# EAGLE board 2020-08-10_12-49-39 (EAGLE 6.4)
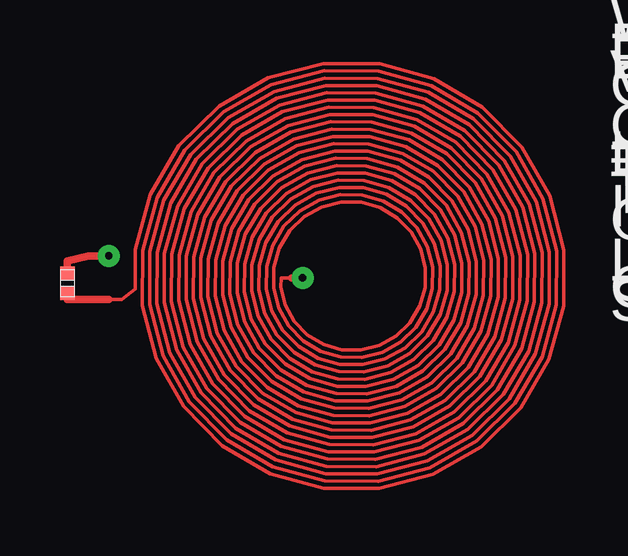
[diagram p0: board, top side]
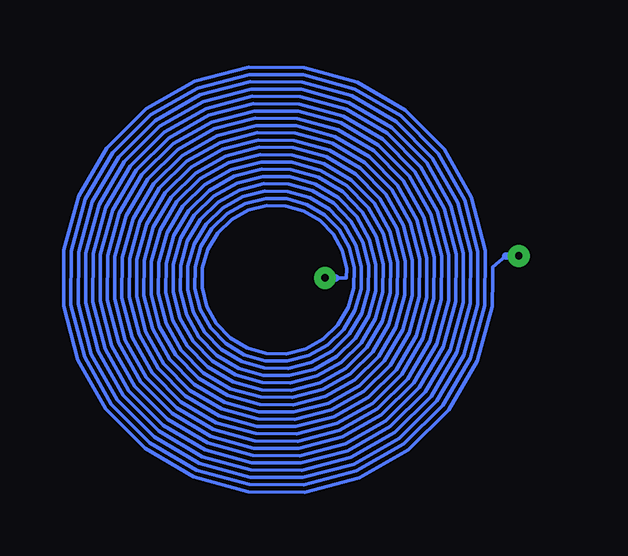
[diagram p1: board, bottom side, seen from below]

No outline drawn. Coordinates in mm, seen from the top.
Copper layers ((1*2)+(15*16)): TOP / INTERNAL1 / layer 15 / BOTTOM

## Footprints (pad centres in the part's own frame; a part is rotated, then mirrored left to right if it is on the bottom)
0402 = smd 0.559 x 0.61: 1 -0.419,0; 2 0.419,0

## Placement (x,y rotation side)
CSensor  [0402]  2.03,12.09 90 top

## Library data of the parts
CSensor = ultra-librarian

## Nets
3: CSensor.1 CSensor.2

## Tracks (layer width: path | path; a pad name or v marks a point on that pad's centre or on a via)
3  (via drill 0.3 pad 0.91)
  TOP 0.152: 11.39,12.32 10.94,12.32 10.93,11.93 11.12,11.18 11.49,10.5 12.04,9.94 12.71,9.53 13.47,9.32 14.26,9.3 15.03,9.5 15.73,9.88 16.31,10.44 16.72,11.13 16.94,11.91 16.95,12.72 16.75,13.51 16.36,14.23 15.79,14.82 15.08,15.24 14.28,15.47 13.45,15.48 12.64,15.28 11.91,14.87 11.3,14.28 10.87,13.56 10.64,12.74 10.62,11.89 10.83,11.06 11.25,10.31 11.85,9.69 12.6,9.25 13.43,9.01 14.3,9 15.15,9.21 15.92,9.64 16.55,10.26 17,11.02 17.25,11.87 17.26,12.76 17.04,13.63 16.6,14.41 15.97,15.06 15.19,15.52 14.32,15.77 13.41,15.78 12.52,15.56 11.72,15.11 11.06,14.47 10.59,13.67 10.33,12.78 10.32,11.85 10.55,10.94 11.01,10.12 11.67,9.45 12.48,8.97 13.39,8.71 14.34,8.7 15.27,8.93 16.1,9.4 16.79,10.07 17.29,10.9 17.55,11.83 17.56,12.8 17.32,13.75 16.84,14.6 16.16,15.3 15.31,15.81 14.36,16.07 13.37,16.09 12.4,15.84 11.53,15.35 10.82,14.65 10.3,13.79 10.03,12.82 10.02,11.81 10.27,10.83 10.77,9.94 11.48,9.21 12.36,8.68 13.35,8.4 14.38,8.39 15.38,8.65 16.29,9.16 17.04,9.88 17.57,10.78 17.85,11.79 17.86,12.84 17.6,13.86 17.09,14.79 16.34,15.55 15.43,16.09 14.4,16.38 13.33,16.39 12.29,16.12 11.35,15.6 10.57,14.84 10.02,13.91 9.73,12.86 9.71,11.77 9.98,10.71 10.52,9.75 11.29,8.96 12.24,8.4 13.31,8.1 14.42,8.09 15.5,8.36 16.48,8.91 17.28,9.7 17.85,10.66 18.16,11.75 18.17,12.88 17.89,13.98 17.33,14.97 16.53,15.79 15.55,16.37 14.44,16.68 13.29,16.7 12.17,16.41 11.16,15.84 10.33,15.03 9.74,14.03 9.42,12.9 9.41,11.73 9.7,10.59 10.28,9.56 11.11,8.72 12.13,8.12 13.27,7.8 14.46,7.78 15.62,8.08 16.66,8.67 17.52,9.51 18.14,10.55 18.46,11.71 18.47,12.92 18.17,14.1 17.57,15.16 16.72,16.03 15.66,16.66 14.48,16.99 13.25,17 12.05,16.69 10.97,16.08 10.09,15.21 9.45,14.14 9.12,12.94 9.11,11.69 9.42,10.47 10.04,9.38 10.92,8.48 12.01,7.83 13.23,7.49 14.5,7.48 15.74,7.8 16.85,8.43 17.77,9.32 18.42,10.43 18.76,11.67 18.78,12.96 18.45,14.22 17.82,15.35 16.9,16.28 15.78,16.94 14.52,17.29 13.21,17.3 11.94,16.97 10.79,16.33 9.84,15.4 9.17,14.26 8.81,12.98 8.8,11.65 9.14,10.36 9.79,9.19 10.73,8.23 11.89,7.55 13.19,7.19 14.54,7.18 15.85,7.51 17.04,8.18 18.01,9.14 18.7,10.31 19.07,11.63 19.08,13 18.74,14.33 18.06,15.53 17.09,16.52 15.9,17.22 14.56,17.59 13.17,17.61 11.82,17.26 10.6,16.57 9.6,15.59 8.89,14.38 8.51,13.02 8.5,11.61 8.85,10.24 9.55,9.01 10.55,7.99 11.77,7.27 13.15,6.89 14.58,6.87 15.97,7.23 17.22,7.94 18.25,8.95 18.98,10.2 19.37,11.59 19.38,13.04 19.02,14.45 18.3,15.72 17.28,16.76 16.02,17.5 14.6,17.9 13.13,17.91 11.7,17.54 10.41,16.81 9.36,15.77 8.61,14.49 8.21,13.06 8.2,11.57 8.57,10.12 9.31,8.82 10.36,7.75 11.66,6.98 13.11,6.58 14.62,6.57 16.09,6.95 17.41,7.7 18.49,8.76 19.27,10.08 19.68,11.55 19.69,13.08 19.3,14.57 18.54,15.91 17.46,17 16.13,17.79 14.64,18.2 13.09,18.21 11.58,17.82 10.23,17.06 9.12,15.96 8.32,14.61 7.9,13.1 7.89,11.53 8.29,10.01 9.06,8.63 10.17,7.5 11.54,6.7 13.07,6.28 14.66,6.27 16.2,6.67 17.6,7.45 18.74,8.58 19.55,9.96 19.98,11.51 19.99,13.12 19.59,14.69 18.79,16.09 17.65,17.25 16.25,18.07 14.68,18.5 13.05,18.52 11.47,18.11 10.04,17.3 8.87,16.15 8.04,14.73 7.6,13.14 7.59,11.49 8,9.89 8.82,8.45 9.99,7.26 11.42,6.42 13.03,5.97 14.7,5.96 16.32,6.38 17.78,7.21 18.98,8.39 19.83,9.84 20.28,11.47 20.3,13.16 19.87,14.8 19.03,16.28 17.84,17.49 16.37,18.36 14.72,18.81 13.01,18.82 11.35,18.39 9.86,17.54 8.63,16.33 7.76,14.85 7.3,13.18 7.28,11.45 7.72,9.77 8.58,8.26 9.8,7.02 11.3,6.13 12.99,5.67 14.74,5.66 16.44,6.1 17.97,6.97 19.22,8.2 20.12,9.73 20.59,11.43 20.6,13.2 20.15,14.92 19.27,16.47 18.02,17.73 16.48,18.64 14.76,19.11 12.97,19.12 11.23,18.67 9.67,17.79 8.39,16.52 7.47,14.96 6.99,13.22 6.98,11.41 7.44,9.65 8.34,8.07 9.61,6.78 11.19,5.85 12.95,5.37 14.78,5.35 16.56,5.82 18.16,6.72 19.47,8.02 20.4,9.61 20.89,11.39 20.9,13.24 20.43,15.04 19.52,16.65 18.21,17.98 16.6,18.92 14.8,19.42 12.93,19.43 11.12,18.96 9.48,18.03 8.14,16.71 7.19,15.08 6.69,13.26 6.68,11.37 7.15,9.54 8.09,7.89 9.43,6.53 11.07,5.57 12.91,5.06 14.82,5.05 16.67,5.53 18.34,6.48 19.71,7.83 20.68,9.49 21.19,11.35 21.21,13.28 20.72,15.15 19.76,16.84 18.4,18.22 16.72,19.2 14.84,19.72 12.89,19.73 11,19.24 9.29,18.27 7.9,16.89 6.91,15.2 6.38,13.3 6.37,11.33 6.87,9.42 7.85,7.7 9.24,6.29 10.95,5.29 12.87,4.76 14.86,4.75 16.79,5.25 18.53,6.24 19.95,7.64 20.97,9.37 21.5,11.31 21.51,13.32 21,15.27 20,17.02 18.58,18.46 16.84,19.49 14.88,20.02 12.85,20.04 10.88,19.52 9.11,18.51 7.66,17.08 6.62,15.31 6.08,13.34 6.07,11.29 6.59,9.3 7.61,7.51 9.05,6.05 10.84,5 12.83,4.46 14.9,4.44 16.91,4.97 18.71,6 20.2,7.46 21.25,9.26 21.8,11.27 21.81,13.36 21.28,15.39 20.25,17.21 18.77,18.71 16.95,19.77 14.92,20.33 12.81,20.34 10.76,19.8 8.92,18.76 7.41,17.27 6.34,15.43 5.78,13.38 5.76,11.25 6.3,9.18 7.36,7.33 8.87,5.8 10.72,4.72 12.79,4.15 14.94,4.14 17.03,4.68 18.9,5.75 20.44,7.27 21.53,9.14 22.11,11.23 22.12,13.4 21.57,15.51 20.49,17.4 18.96,18.95 17.07,20.05 14.96,20.63 12.77,20.64 10.65,20.09 8.74,19 7.17,17.45 6.06,15.55 5.47,13.42 5.46,11.21 6.02,9.07 7.12,7.14 8.68,5.56 10.6,4.44 12.75,3.85 14.98,3.83 17.14,4.4 19.09,5.51 20.68,7.08 21.82,9.02 22.41,11.19 22.42,13.44 21.85,15.62 20.73,17.59 19.14,19.19 17.19,20.34 15,20.93 12.73,20.95 10.53,20.37 8.55,19.24 6.93,17.64 5.77,15.67 5.17,13.46 5.16,11.17 5.74,8.95 6.88,6.95 8.49,5.32 10.48,4.15 12.71,3.54 15.02,3.53 17.26,4.12 19.27,5.27 20.93,6.9 22.1,8.9 22.71,11.15 22.73,13.48 22.13,15.74 20.98,17.77 19.33,19.44 17.3,20.62 15.04,21.24 12.69,21.25 10.41,20.65 8.36,19.49 6.68,17.83 5.49,15.78 4.87,13.5 4.85,12.32 4.85,11.86 4.31,11.4 3.76,11.4
  TOP 0.304: 11.39,12.32 v11.84,12.32 | v3.76,13.23 2.9,13.23 2.03,13.01 2.03,12.8 | 3.76,11.4 2.9,11.4 2.03,11.4
  BOTTOM 0.152: 11.39,12.32 10.94,12.32 10.93,12.7 11.12,13.45 11.49,14.13 12.04,14.7 12.71,15.1 13.47,15.31 14.26,15.33 15.03,15.13 15.73,14.75 16.31,14.19 16.72,13.5 16.94,12.72 16.95,11.91 16.75,11.12 16.36,10.4 15.79,9.81 15.08,9.39 14.28,9.16 13.45,9.15 12.64,9.36 11.91,9.76 11.3,10.35 10.87,11.07 10.64,11.89 10.62,12.74 10.83,13.57 11.25,14.32 11.85,14.94 12.6,15.38 13.43,15.62 14.3,15.63 15.15,15.42 15.92,14.99 16.55,14.38 17,13.62 17.25,12.76 17.26,11.87 17.04,11 16.6,10.22 15.97,9.57 15.19,9.11 14.32,8.86 13.41,8.85 12.52,9.07 11.72,9.52 11.06,10.16 10.59,10.96 10.33,11.85 10.32,12.78 10.55,13.69 11.01,14.51 11.67,15.18 12.48,15.66 13.39,15.92 14.34,15.94 15.27,15.7 16.1,15.23 16.79,14.56 17.29,13.73 17.55,12.8 17.56,11.83 17.32,10.88 16.84,10.03 16.16,9.33 15.31,8.82 14.36,8.56 13.37,8.54 12.4,8.79 11.53,9.28 10.82,9.98 10.3,10.84 10.03,11.81 10.02,12.82 10.27,13.81 10.77,14.69 11.48,15.43 12.36,15.95 13.35,16.23 14.38,16.24 15.38,15.98 16.29,15.48 17.04,14.75 17.57,13.85 17.85,12.84 17.86,11.79 17.6,10.77 17.09,9.84 16.34,9.09 15.43,8.54 14.4,8.25 13.33,8.24 12.29,8.51 11.35,9.03 10.57,9.79 10.02,10.72 9.73,11.77 9.71,12.86 9.98,13.92 10.52,14.88 11.29,15.67 12.24,16.23 13.31,16.53 14.42,16.54 15.5,16.27 16.48,15.72 17.28,14.94 17.85,13.97 18.16,12.88 18.17,11.75 17.89,10.65 17.33,9.66 16.53,8.84 15.55,8.26 14.44,7.95 13.29,7.94 12.17,8.22 11.16,8.79 10.33,9.6 9.74,10.61 9.42,11.73 9.41,12.9 9.7,14.04 10.28,15.07 11.11,15.91 12.13,16.51 13.27,16.83 14.46,16.85 15.62,16.55 16.66,15.96 17.52,15.12 18.14,14.08 18.46,12.92 18.47,11.71 18.17,10.53 17.57,9.47 16.72,8.6 15.66,7.97 14.48,7.64 13.25,7.63 12.05,7.94 10.97,8.55 10.09,9.42 9.45,10.49 9.12,11.69 9.11,12.94 9.42,14.16 10.04,15.25 10.92,16.15 12.01,16.8 13.23,17.14 14.5,17.15 15.74,16.83 16.85,16.2 17.77,15.31 18.42,14.2 18.76,12.96 18.78,11.67 18.45,10.41 17.82,9.29 16.9,8.36 15.78,7.69 14.52,7.34 13.21,7.33 11.94,7.66 10.79,8.3 9.84,9.23 9.17,10.37 8.81,11.65 8.8,12.98 9.14,14.28 9.79,15.44 10.73,16.4 11.89,17.08 13.19,17.44 14.54,17.45 15.85,17.12 17.04,16.45 18.01,15.49 18.7,14.32 19.07,13 19.08,11.63 18.74,10.3 18.06,9.1 17.09,8.11 15.9,7.41 14.56,7.04 13.17,7.03 11.82,7.37 10.6,8.06 9.6,9.04 8.89,10.25 8.51,11.61 8.5,13.02 8.85,14.39 9.55,15.63 10.55,16.64 11.77,17.36 13.15,17.75 14.58,17.76 15.97,17.4 17.22,16.69 18.25,15.68 18.98,14.44 19.37,13.04 19.38,11.59 19.02,10.18 18.3,8.91 17.28,7.87 16.02,7.13 14.6,6.73 13.13,6.72 11.7,7.09 10.41,7.82 9.36,8.86 8.61,10.14 8.21,11.57 8.2,13.06 8.57,14.51 9.31,15.81 10.36,16.88 11.66,17.65 13.11,18.05 14.62,18.06 16.09,17.68 17.41,16.93 18.49,15.87 19.27,14.55 19.68,13.08 19.69,11.55 19.3,10.06 18.54,8.72 17.46,7.63 16.13,6.84 14.64,6.43 13.09,6.42 11.58,6.81 10.23,7.58 9.12,8.67 8.32,10.02 7.9,11.53 7.89,13.1 8.29,14.63 9.06,16 10.17,17.13 11.54,17.93 13.07,18.35 14.66,18.37 16.2,17.96 17.6,17.18 18.74,16.05 19.55,14.67 19.98,13.12 19.99,11.51 19.59,9.95 18.79,8.54 17.65,7.38 16.25,6.56 14.68,6.13 13.05,6.11 11.47,6.52 10.04,7.33 8.87,8.48 8.04,9.9 7.6,11.49 7.59,13.14 8,14.74 8.82,16.19 9.99,17.37 11.42,18.21 13.03,18.66 14.7,18.67 16.32,18.25 17.78,17.42 18.98,16.24 19.83,14.79 20.28,13.16 20.3,11.47 19.87,9.83 19.03,8.35 17.84,7.14 16.37,6.28 14.72,5.82 13.01,5.81 11.35,6.24 9.86,7.09 8.63,8.3 7.76,9.79 7.3,11.45 7.28,13.18 7.72,14.86 8.58,16.37 9.8,17.61 11.3,18.5 12.99,18.96 14.74,18.97 16.44,18.53 17.97,17.66 19.22,16.43 20.12,14.9 20.59,13.2 20.6,11.43 20.15,9.71 19.27,8.16 18.02,6.9 16.48,5.99 14.76,5.52 12.97,5.51 11.23,5.96 9.67,6.85 8.39,8.11 7.47,9.67 6.99,11.41 6.98,13.22 7.44,14.98 8.34,16.56 9.61,17.86 11.19,18.78 12.95,19.26 14.78,19.28 16.56,18.81 18.16,17.91 19.47,16.61 20.4,15.02 20.89,13.24 20.9,11.39 20.43,9.59 19.52,7.98 18.21,6.65 16.6,5.71 14.8,5.21 12.93,5.2 11.12,5.67 9.48,6.6 8.14,7.92 7.19,9.55 6.69,11.37 6.68,13.26 7.15,15.1 8.09,16.75 9.43,18.1 11.07,19.06 12.91,19.57 14.82,19.58 16.67,19.1 18.34,18.15 19.71,16.8 20.68,15.14 21.19,13.28 21.21,11.35 20.72,9.48 19.76,7.79 18.4,6.41 16.72,5.43 14.84,4.91 12.89,4.9 11,5.39 9.29,6.36 7.9,7.74 6.91,9.43 6.38,11.33 6.37,13.3 6.87,15.21 7.85,16.93 9.24,18.34 10.95,19.34 12.87,19.87 14.86,19.89 16.79,19.38 18.53,18.39 19.95,16.99 20.97,15.26 21.5,13.32 21.51,11.31 21,9.36 20,7.61 18.58,6.17 16.84,5.14 14.88,4.61 12.85,4.59 10.88,5.11 9.11,6.12 7.66,7.55 6.62,9.32 6.08,11.29 6.07,13.34 6.59,15.33 7.61,17.12 9.05,18.59 10.84,19.63 12.83,20.18 14.9,20.19 16.91,19.66 18.71,18.64 20.2,17.17 21.25,15.37 21.8,13.36 21.81,11.27 21.28,9.24 20.25,7.42 18.77,5.92 16.95,4.86 14.92,4.3 12.81,4.29 10.76,4.83 8.92,5.87 7.41,7.37 6.34,9.2 5.78,11.25 5.76,13.38 6.3,15.45 7.36,17.3 8.87,18.83 10.72,19.91 12.79,20.48 14.94,20.49 17.03,19.95 18.9,18.88 20.44,17.36 21.53,15.49 22.11,13.4 22.12,11.23 21.57,9.12 20.49,7.23 18.96,5.68 17.07,4.58 14.96,4 12.77,3.99 10.65,4.54 8.74,5.63 7.17,7.18 6.06,9.08 5.47,11.21 5.46,13.42 6.02,15.56 7.12,17.49 8.68,19.07 10.6,20.2 12.75,20.78 14.98,20.8 17.14,20.23 19.09,19.12 20.68,17.55 21.82,15.61 22.41,13.44 22.42,11.19 21.85,9.01 20.73,7.05 19.14,5.44 17.19,4.29 15,3.7 12.73,3.68 10.53,4.26 8.55,5.39 6.93,6.99 5.77,8.96 5.17,11.17 5.16,13.46 5.74,15.68 6.88,17.68 8.49,19.31 10.48,20.48 12.71,21.09 15.02,21.1 17.26,20.51 19.27,19.36 20.93,17.73 22.1,15.73 22.71,13.48 22.73,11.15 22.13,8.89 20.98,6.86 19.33,5.2 17.3,4.01 15.04,3.39 12.69,3.38 10.41,3.98 8.36,5.14 6.68,6.8 5.49,8.85 4.87,11.13 4.85,12.32 4.85,12.77 4.31,13.23
  BOTTOM 0.304: 11.39,12.32 v11.84,12.32 | 4.31,13.23 v3.76,13.23

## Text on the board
ASSYNOTES: Exported from WEBENCH Coil Designer Tool | ------------------------- | WEBENCH Design Information | Design Id - 2 | Exported on - 2020/08/10 12:49:36 | Customized for LDC1614 | Version - 1.1 | Coil Parameters | -------------- | Layers = 2 | Trace Width = 5.98 mils | Turns = 20 | Trace Spacing = 5.98 mils | Inner Diameter = 231 mils (Approx.) | Outer Diameter = 710 mils (Approx.) | ------------------------- | Layer Stack Information | Copper thickness = 1.0 Oz-Cu | Space between TOP and BOTTOM = 4.0 mils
